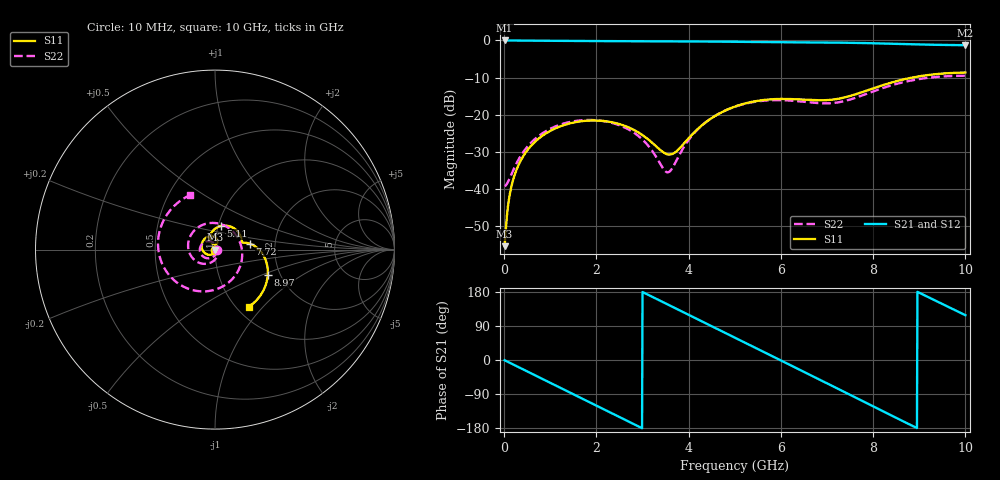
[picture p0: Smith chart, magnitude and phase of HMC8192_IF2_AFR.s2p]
! Analog Devices, Inc.
! 1 Analog Way
! Wilmington, MA 01887
! http://www.analog.com
! Date:  2021-09-17 NN
! Board Name:  EVALHMC8192LG Revision A with HMC8192LG installed
! File Description:  Automatic Fixture Removal S-Parameters for IF2 Port connector and board loss de-embedding
! File Generation:  Calibrated Network Analyzer
! Chip Part Number:  HMC8192
! Chip Description:  Wideband IQ Mixer
! Chip Frequency:  20 to 42 GHz
! Chip Package:  LGA_CAV, 4 x 4 x 1.55 mm
! IF2 Port:  HMC8192LG removed and end of trace left open
! Note:
!  Analog Devices supplies this data as a sample of measured data at the evaluation board
!  ports for this product.  Your particular data for this product may vary.
!  Analog Devices reserves the right to change this data at anytime.
!  All lines below in this file are as is from the Network Analyzer.
!Agilent Technologies,N5245A,MY52451809,A.10.47.06
!Automatic Fixture Removal (AFR)
!Date: Friday, September 17, 2021 2:57:52 AM
!S2P File: Measurements: S11,S21,S12,S22:
# MHz S  RI  R 50
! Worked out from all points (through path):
!   1000 points, 10 MHz to 10 GHz, reference 50 ohm
!   highest |S21| = 0.01 dB at 10 MHz (marker M1); lowest = -1.3 dB at 10 GHz (marker M2)
!   group delay of S21, straight-line fit = 167 ps
!   lowest |S11| = -55.5 dB at 10 MHz (marker M3), VSWR 1.00, Z = 50.2 - j0.0699 ohm
!   |S11| at or under -10 dB: start of sweep to 8.85 GHz
!   |S22| runs from -39.3 to -9.5 dB; largest |S21 - S12| = 1.5e-15
!   S11 on the Smith chart (normalised r, x): 10 MHz: 1.00, -0.00; 5.11 GHz: 1.03, +0.27; 7.72 GHz: 1.48, +0.10; 8.97 GHz: 1.72, -0.54; 10 GHz: 1.14, -0.84
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10  0.00153 -0.000697  1.001 -0.0106  1.001 -0.0106  0.0108 -0.000819
170  -0.00111 -0.0115  0.983 -0.1781  0.983 -0.1781  0.00882 -0.0137
440  -0.0144 -0.0253  0.8909 -0.4456  0.8909 -0.4456  -0.00194 -0.0328
1090  -0.0629 -0.0132  0.4064 -0.9018  0.4064 -0.9018  -0.0499 -0.0467
1680  -0.0708 0.0404  -0.191 -0.9651  -0.191 -0.9651  -0.0824 -0.0157
2100  -0.0441 0.0699  -0.5823 -0.7896  -0.5823 -0.7896  -0.0809 0.017
2570  -0.00461 0.072  -0.885 -0.4192  -0.885 -0.4192  -0.0538 0.043
2960  0.0138 0.0532  -0.9778 -0.0318  -0.9778 -0.0318  -0.0205 0.0439
3340  0.0101 0.0338  -0.9117 0.3514  -0.9117 0.3514  0.00767 0.0229
3590  -0.00152 0.0289  -0.7876 0.5762  -0.7876 0.5762  0.0171 -0.000651
4210  -0.0279 0.0587  -0.2724 0.9313  -0.2724 0.9313  -0.00909 -0.0638
4600  -0.0184 0.0963  0.1216 0.9574  0.1216 0.9574  -0.0581 -0.0796
5010  0.0194 0.1272  0.5068 0.8139  0.5068 0.8139  -0.1148 -0.0574
5110  0.0317 0.1312  0.5881 0.7552  0.5881 0.7552  -0.1262 -0.0457
5900  0.123 0.1056  0.9431 0.0787  0.9431 0.0787  -0.1274 0.0916
6670  0.1489 0.0495  0.7041 -0.6242  0.7041 -0.6242  0.0354 0.1408
7210  0.1575 0.0388  0.2523 -0.9012  0.2523 -0.9012  0.141 0.0351
7720  0.1941 0.0329  -0.2471 -0.8922  -0.2471 -0.8922  0.1245 -0.1263
8340  0.2634 -0.0219  -0.7248 -0.5441  -0.7248 -0.5441  -0.0667 -0.2329
8970  0.2941 -0.1412  -0.8846 0.0119  -0.8846 0.0119  -0.2802 -0.1069
9440  0.2647 -0.2368  -0.7662 0.4175  -0.7662 0.4175  -0.3097 0.0983
10000  0.189 -0.3181  -0.4088 0.7618  -0.4088 0.7618  -0.1373 0.3049
